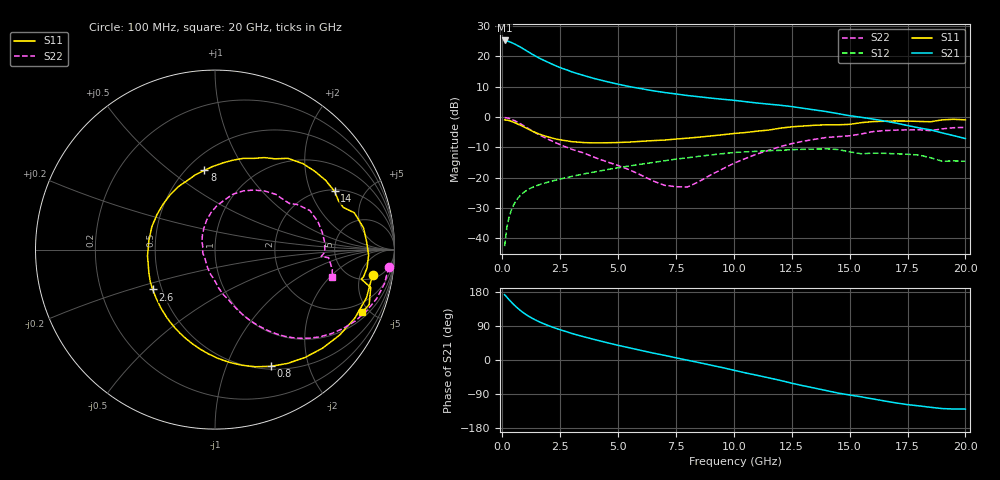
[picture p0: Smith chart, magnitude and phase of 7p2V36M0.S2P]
! Infineon Technologies  Discrete & RF Semiconductors
! bfp620
! VCE =  2.3 V,  IC =  6.0 mA
! Common Emitter S-Parameters:  Sep 2002
# GHz  S  MA  R  50
!  f  S11  S21  S12  S22
! GHz  MAG  ANG  MAG  ANG  MAG  ANG  MAG  ANG
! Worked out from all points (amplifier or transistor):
!   59 points, 100 MHz to 20 GHz, reference 50 ohm
!   highest |S21| = 25.2 dB at 100 MHz (marker M1)
!   |S21| within 3 dB of that: start of sweep to 959.8 MHz
!   unconditionally stable (mu >= 1): 4.549 GHz to 11.54 GHz; 14.83 GHz to 15.18 GHz; 17.19 GHz to end of sweep
!   at 1 GHz: K = 0.37, MSG = 23.2 dB, |S12| = -24.5 dB
!   at 5.5 GHz: K = 1.05, MAG = 11.7 dB, |S12| = -16.2 dB
!   at 20 GHz: K = 1.31, MAG = 0.4 dB, |S12| = -14.6 dB
!   S11 on the Smith chart (normalised r, x): 100 MHz: 6, -8; 800 MHz: 0.54, -1.45; 2.6 GHz: 0.45, -0.24; 8 GHz: 0.61, +0.67; 14 GHz: 2.08, +2.99; 20 GHz: 1.33, -4.54
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0.1  0.8894 -9.1  18.16 172.4  0.0074 72.7  0.9734 -5.7
0.2  0.8856 -17.7  17.86 165.5  0.0154 75.2  0.9631 -11.4
0.3  0.8673 -26.2  17.36 158.7  0.0229 72.8  0.9405 -17.0
0.4  0.8418 -34.5  16.75 152.2  0.0298 69.6  0.9104 -22.2
0.5  0.8129 -42.5  16.09 146.0  0.0361 66.3  0.8758 -27.1
0.6  0.7826 -50.2  15.39 140.2  0.0418 63.1  0.8386 -31.6
0.8  0.7211 -64.4  13.98 129.8  0.0516 57.3  0.7615 -39.6
1.1  0.6326 -82.9  11.93 116.9  0.063 50.4  0.6505 -48.9
1.3  0.5813 -93.8  10.74 109.8  0.0689 46.9  0.5855 -53.6
1.5  0.5388 -103.7  9.728 103.6  0.0739 44.2  0.5297 -57.5
1.7  0.5047 -112.8  8.891 98.0  0.0784 42.0  0.4828 -60.7
2  0.4647 -125.2  7.859 90.6  0.0846 39.5  0.4249 -64.7
2.6  0.4123 -147.4  6.274 77.8  0.0965 35.5  0.3358 -71.1
3.5  0.3776 -174.8  4.828 61.6  0.1145 30.2  0.2551 -79.4
5  0.3777 148.6  3.456 38.7  0.1449 21.1  0.158 -94.0
7  0.4146 111.8  2.522 12.4  0.1888 7.2  0.0746 -138.8
8  0.4458 97.6  2.247 -0.6  0.2116 -1.4  0.0699 167.0
10.5  0.5519 67.0  1.781 -34.0  0.2651 -26.7  0.2061 96.4
13.5  0.7273 32.0  1.3 -74.3  0.2937 -58.2  0.4277 49.7
14  0.741 26.0  1.222 -80.8  0.2976 -64.6  0.4578 42.3
17  0.8565 -2.1  0.791 -113.2  0.2464 -89.1  0.6052 9.3
20  0.8919 -23.0  0.439 -129.5  0.1857 -102.2  0.6704 -13.3
